(* Logix 5000 AddOnInstructionDefinition export AMCI_SD4840E2_Program_Motor_Current; software revision 20.03 *)

ADD_ON_INSTRUCTION AMCI_SD4840E2_Program_Motor_Current   (* revision 1.0, vendor AMCI *)
VAR_INPUT
   Motor_Current : INT; {required}
END_VAR
VAR_IN_OUT
   AMCI_SD4840E2_output_data : _000A:SD4840E2_4342D302:O:0; {required}
END_VAR
VAR
   Upper_Result_X_1000 : DINT;
   command_data_block : INT[10];
        [0]   // Command Bits MSW
        [1]   // Command Bits LSW
        [2]   // Upper Target Position
        [3]   // Lower Target Position
        [4]   // Upper Programmed Speed
        [5]   // Lower Programmed Speed
END_VAR

ROUTINE Logic   (* ladder *)
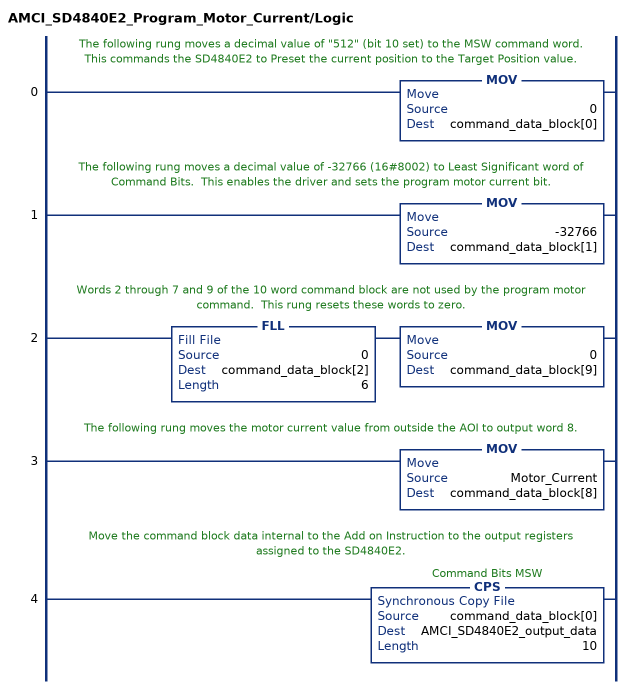
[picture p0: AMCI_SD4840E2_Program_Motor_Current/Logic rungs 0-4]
   // The following rung moves a decimal value of "512" (bit 10 set) to the MSW command word.  This commands the SD4840E2 to Preset the current position to the Target Position value.
   0: MOV(0,command_data_block[0]);
   // The following rung moves a decimal value of -32766 (16#8002) to Least Significant word of Command Bits.  This enables the driver and sets the program motor current bit.
   1: MOV(-32766,command_data_block[1]);
   // Words 2 through 7 and 9 of the 10 word command block are not used by the program motor command.  This rung resets these words to zero.
   2: FLL(0,command_data_block[2],6)MOV(0,command_data_block[9]);
   // The following rung moves the motor current value from outside the AOI to output word 8.
   3: MOV(Motor_Current,command_data_block[8]);
   // Move the command block data internal to the Add on Instruction to the output registers assigned to the SD4840E2.
   4: CPS(command_data_block[0],AMCI_SD4840E2_output_data,10);
END_ROUTINE
END_ADD_ON_INSTRUCTION
